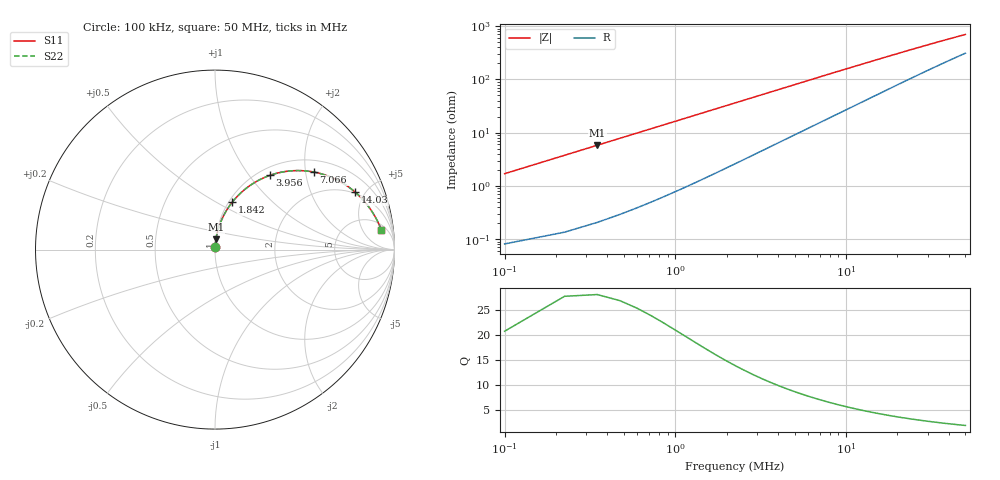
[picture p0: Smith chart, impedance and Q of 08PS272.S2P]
! Coilcraft 0805PS-272 Power Chip Inductor
! 5 February 2003
# MHZ S MA R 50
!Freq  MagS11  AngS11  MagS21  AngS21  MagS12  AngS12  MagS22  AngS22
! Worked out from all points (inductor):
!   403 points, 100 kHz to 50 MHz, reference 50 ohm
!   read as one part in series: L = 2.64 uH near 348.8 kHz
!   highest Q = 23.9 at 348.8 kHz (marker M1), where L = 2.65 uH
!   S11 on the Smith chart (normalised r, x): 100 kHz: 1.00, +0.03; 1.842 MHz: 1.04, +0.60; 3.956 MHz: 1.13, +1.27; 7.066 MHz: 1.31, +2.22; 14.03 MHz: 1.91, +4.26; 50 MHz: 7, +12
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0.1  0.01697 86.3  0.999 -1.0  0.999 -1.0  0.01697 86.3
0.2244  0.03758 85.8  0.9979 -2.2  0.9979 -2.2  0.03758 85.8
0.3488  0.05795 84.6  0.9963 -3.3  0.9963 -3.3  0.05795 84.6
0.4732  0.0781 83.4  0.994 -4.5  0.994 -4.5  0.0781 83.4
0.5976  0.09805 82.1  0.9913 -5.6  0.9913 -5.6  0.09805 82.1
0.8464  0.1373 79.6  0.9845 -7.9  0.9845 -7.9  0.1373 79.6
1.2196  0.1941 75.8  0.9709 -11.2  0.9709 -11.2  0.1941 75.8
1.4684  0.2306 73.4  0.96 -13.3  0.96 -13.3  0.2306 73.4
1.8416  0.2826 69.9  0.9413 -16.4  0.9413 -16.4  0.2826 69.9
2.2148  0.3314 66.6  0.9202 -19.3  0.9202 -19.3  0.3314 66.6
2.7124  0.3912 62.5  0.8897 -23.0  0.8897 -23.0  0.3912 62.5
3.9564  0.5147 53.5  0.8079 -30.8  0.8079 -30.8  0.5147 53.5
5.3248  0.6138 45.7  0.7204 -37.6  0.7204 -37.6  0.6138 45.7
7.0664  0.7 38.1  0.6233 -43.9  0.6233 -43.9  0.7 38.1
8.4348  0.7466 33.6  0.5598 -47.5  0.5598 -47.5  0.7466 33.6
10.9228  0.8028 27.5  0.4687 -52.2  0.4687 -52.2  0.8028 27.5
14.0328  0.8443 22.3  0.3874 -55.6  0.3874 -55.6  0.8443 22.3
16.7696  0.8669 19.0  0.3356 -57.5  0.3356 -57.5  0.8669 19.0
25.1044  0.9024 13.2  0.2392 -59.5  0.2392 -59.5  0.9024 13.2
33.4392  0.9184 10.1  0.1873 -59.2  0.1873 -59.2  0.9184 10.1
41.774  0.9274 8.2  0.1553 -58.1  0.1553 -58.1  0.9274 8.2
50  0.9332 6.9  0.1338 -56.7  0.1338 -56.7  0.9332 6.9
